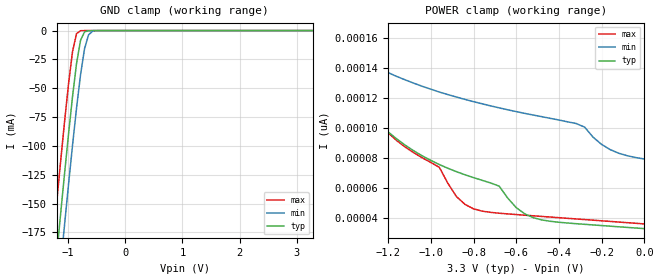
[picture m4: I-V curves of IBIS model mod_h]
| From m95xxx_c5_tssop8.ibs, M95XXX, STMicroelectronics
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|   Model mod_h
[Model]   mod_h
Model_type Input
Vinl   =   0.825V
Vinh   =   2.475V
C_comp   2.119pF   2.024pF   2.324pF
[Temperature Range]  25.0000   85.0000   -40.0000
[Voltage Range]   3.3000V   2.7000V   3.6000V
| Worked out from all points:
|   GND clamp passes 1 mA (typ) near -0.70 V on its own axis
[GND_clamp]
|Voltage   I(typ)   I(min)   I(max)
-3.3V     -1.355A    -1.397A    -1.313A
-1.27V    -233mA     -277.9mA   -187.4mA
-1.2V     -196.1mA   -241mA     -150.5mA
-1.13V    -159.7mA   -204.5mA   -114.2mA
-1.06V    -124.1mA   -168.5mA   -79.16mA
-920mV    -57.12mA   -99.32mA   -18.15mA
-850mV    -28.51mA   -67.14mA   -2.609mA
-780mV    -8.357mA   -38.23mA   -131.1uA
-710mV    -1.089mA   -15.64mA   -5.451uA
-640mV    -95.71uA   -3.67mA    -224.5nA
-570mV    -7.943uA   -542uA     -9.245nA
3.28V     6.871pA    47.88pA    6.69pA
[POWER_clamp]
|Voltage   I(typ)   I(min)   I(max)
-3.28V    711.2nA    8.459nA    1.989uA
-1.56V    175.5pA    171.2pA    199.3pA
-1.52V    162.2pA    165.9pA    179.8pA
-1.48V    150.4pA    161.2pA    163.2pA
-1.28V    108.5pA    142.5pA    109.2pA
-960mV    75.69pA    123.9pA    73.84pA
-840mV    68.9pA     119pA      49.21pA
-680mV    61.34pA    113.4pA    43.33pA
-520mV    40.36pA    108.6pA    41.6pA
-320mV    36.37pA    103pA      39.53pA
-160mV    34.71pA    85.61pA    37.87pA
0V        33.08pA    79.36pA    36.22pA
